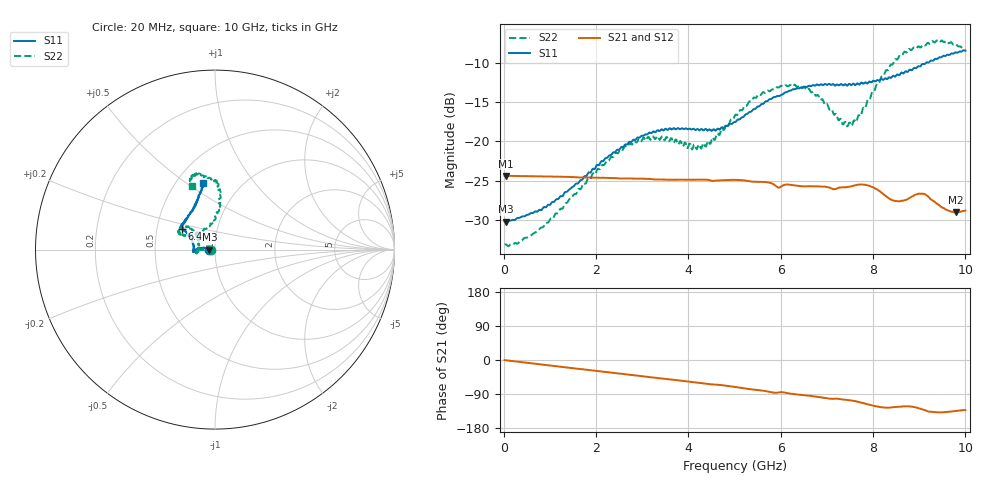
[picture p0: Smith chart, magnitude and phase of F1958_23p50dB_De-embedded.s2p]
! Integrated Device Technology
! Corporate Headquarters
! 6024 Silver Creek Valley Road
! San Jose, CA 95138  USA
! Phone:  1-408-284-8200
! Toll Free:  1-800-223-1366
! Webpage:  http://www.idt.com/
! Timing and RF Division
! 515 Groton Road, Suite 102
! Westford, MA 01886-6024
! Device:  F1958
! Description: 7-bit 0.25 dB Digital Step Attenuator
! Frequency:  0.001 -  6.000 GHz
! Package:  4x4 mm Thin QFN Plastic Package: 24 pin
! Ports:  2 RF, 12 DC
!  Pin  1  = D0
!  Pin  2  = VDD
!  Pin  3  = VMODE
!  Pin  4  = GND
!  Pin  5  = RF1  =  Port 1
!  Pin  6  = GND
!  Pin  7  = GND
!  Pin  8  = GND
!  Pin  9  = GND
!  Pin 10  = GND
!  Pin 11  = GND
!  Pin 12  = GND
!  Pin 13  = GND
!  Pin 14  = RF2  =  Port 2
!  Pin 15  = GND
!  Pin 16  = LE
!  Pin 17  = CLK
!  Pin 18  = DATA
!  Pin 19  = D6
!  Pin 20  = D5
!  Pin 21  = D4
!  Pin 22  = D3
!  Pin 23  = D2
!  Pin 24  = D1
! State:  94
! Atten State:  23.50 dB
! Voltage:  +3.30 Volts
! Current:  0.257 mA
! Data:  The device was measured on a F1958 evaluation board which has
!  individual transmission lines to the RF pins.  Data was collected
!  using a calibrated network analyzer.  The evaluation board was
!  de-embedded using Automatic Fixture Removal (AFR).
!  The reference plane is the edge of the package pin.
! Misc:
!  Action Tracker AT0419
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# GHz S dB R 50
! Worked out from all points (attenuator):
!   500 points, 20 MHz to 10 GHz, reference 50 ohm
!   highest |S21| = -24.37 dB at 40 MHz (marker M1); lowest = -29.0 dB at 9.8 GHz (marker M2)
!   lowest |S11| = -30.2 dB at 40 MHz (marker M3), VSWR 1.06, Z = 47 - j0.0428 ohm
!   |S11| at or under -10 dB: start of sweep to 9.151 GHz
!   |S22| runs from -33.3 to -7.2 dB; largest |S21 - S12| = 0.0003
!   S11 on the Smith chart (normalised r, x): 20 MHz: 0.94, -0.00; 6.4 GHz: 0.67, +0.16; 10 GHz: 0.67, +0.58
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0.02  -30.15 -179.0  -24.37 -0.3  -24.36 -0.3  -33.10 -178.3
0.04  -30.18 -179.2  -24.37 -0.6  -24.36 -0.6  -33.05 -177.4
0.72  -28.94 172.5  -24.42 -10.5  -24.41 -10.5  -31.40 178.1
1.7  -24.87 170.7  -24.57 -24.4  -24.56 -24.3  -25.64 177.5
2.6  -20.63 176.7  -24.70 -37.1  -24.67 -37.1  -20.82 -177.2
3.36  -18.66 -175.7  -24.82 -48.0  -24.83 -48.1  -19.62 -168.5
4.24  -18.59 -179.0  -24.85 -60.1  -24.87 -60.2  -20.43 169.8
4.52  -18.59 174.0  -25.01 -64.3  -25.02 -64.3  -19.49 154.4
5.02  -17.53 160.8  -24.88 -71.4  -24.89 -71.3  -16.60 139.9
5.6  -15.23 150.9  -25.15 -80.6  -25.15 -80.6  -13.83 140.4
6.4  -13.26 148.0  -25.66 -91.8  -25.68 -91.7  -12.87 154.0
6.68  -12.90 146.9  -25.69 -95.3  -25.70 -95.2  -13.74 155.1
7.32  -12.72 141.7  -25.84 -103.8  -25.85 -103.8  -17.43 135.4
7.5  -12.73 138.6  -25.73 -106.3  -25.73 -106.2  -17.60 117.5
7.68  -12.69 135.7  -25.47 -110.4  -25.47 -110.3  -16.70 99.9
7.92  -12.38 129.4  -25.63 -118.1  -25.63 -118.1  -14.70 89.2
8.34  -11.87 119.4  -27.20 -125.7  -27.20 -125.8  -10.79 83.9
8.66  -11.37 113.7  -27.49 -122.4  -27.52 -122.5  -8.75 86.9
9.1  -10.18 107.7  -26.64 -131.5  -26.65 -131.7  -7.72 98.6
9.5  -9.21 101.8  -28.40 -138.1  -28.41 -138.1  -7.20 106.2
9.8  -8.69 101.1  -29.01 -134.4  -29.02 -134.4  -7.65 109.7
10  -8.48 100.2  -28.77 -132.3  -28.79 -132.1  -8.42 110.2
